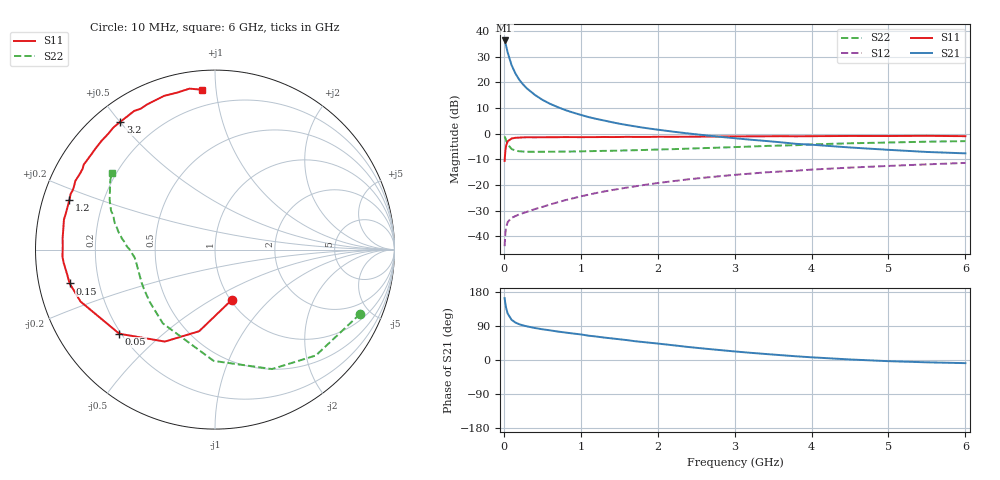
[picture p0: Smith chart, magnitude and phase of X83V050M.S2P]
! SIEMENS Small Signal Semiconductors
! BFP136W
! Si NPN RF Bipolar Junction Transistor in SOT343
! VCE = 3 V  IC = 50 mA
! Common Emitter S-Parameters:  September  1994
# GHz  S  MA  R  50
!  f  S11  S21  S12  S22
! GHz  MAG  ANG  MAG  ANG  MAG  ANG  MAG  ANG
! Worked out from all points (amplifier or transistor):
!   40 points, 10 MHz to 6 GHz, reference 50 ohm
!   highest |S21| = 36.4 dB at 10 MHz (marker M1)
!   |S21| within 3 dB of that: start of sweep to 36.57 MHz
!   unconditionally stable (mu >= 1): 643.6 MHz to 2.88 GHz
!   at 200 MHz: K = 0.55, MSG = 26.3 dB, |S12| = -31.5 dB
!   at 1.5 GHz: K = 1.12, MAG = 10.6 dB, |S12| = -21.5 dB
!   at 6 GHz: K = 0.96, MSG = 1.9 dB, |S12| = -11.4 dB
!   S11 on the Smith chart (normalised r, x): 10 MHz: 1.02, -0.62; 50 MHz: 0.19, -0.36; 150 MHz: 0.09, -0.11; 1.2 GHz: 0.08, +0.17; 3.2 GHz: 0.08, +0.50; 6 GHz: 0.10, +0.92
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0.01  0.2941 -71.1  65.72 163.2  0.0064 73.4  0.8846 -23.9
0.02  0.4633 -101.0  58.51 148.6  0.0116 60.7  0.8147 -46.4
0.03  0.5837 -118.6  51.25 137.3  0.015 53.5  0.7373 -64.5
0.05  0.7102 -138.7  38.19 122.5  0.0189 40.3  0.6202 -90.7
0.1  0.8033 -158.9  21.82 106.2  0.0228 32.9  0.5033 -125.3
0.15  0.8315 -166.9  14.97 98.9  0.0247 33.0  0.4661 -141.2
0.2  0.8373 -171.6  11.28 94.4  0.0267 33.9  0.4536 -150.2
0.25  0.8461 -174.9  9.118 91.2  0.0282 35.9  0.4483 -155.9
0.3  0.8507 -177.3  7.626 88.8  0.0299 38.4  0.4444 -159.8
0.4  0.8486 178.7  5.751 84.6  0.0337 43.4  0.443 -164.9
0.5  0.8514 175.7  4.583 81.1  0.0373 46.0  0.4432 -168.1
0.6  0.8521 173.3  3.825 78.3  0.0415 48.9  0.4444 -170.1
0.7  0.8545 171.0  3.298 75.1  0.0459 51.6  0.446 -171.6
0.9  0.8559 167.1  2.576 69.9  0.0549 54.3  0.4492 -174.1
1.1  0.8558 162.7  2.107 64.2  0.0645 56.0  0.4553 -175.7
1.2  0.8571 161.1  1.945 62.0  0.0696 56.6  0.4588 -176.3
1.7  0.8643 151.9  1.392 49.7  0.0936 56.5  0.4759 179.9
2.2  0.8693 143.6  1.094 38.9  0.1186 54.1  0.4991 176.4
3.2  0.8863 126.5  0.764 19.1  0.1662 46.1  0.5601 167.4
4.5  0.9022 108.3  0.538 1.4  0.218 34.3  0.6492 154.7
5.5  0.908 99.0  0.44 -6.1  0.2521 26.3  0.6974 146.9
6  0.8933 94.5  0.413 -8.3  0.2689 21.9  0.715 143.6
